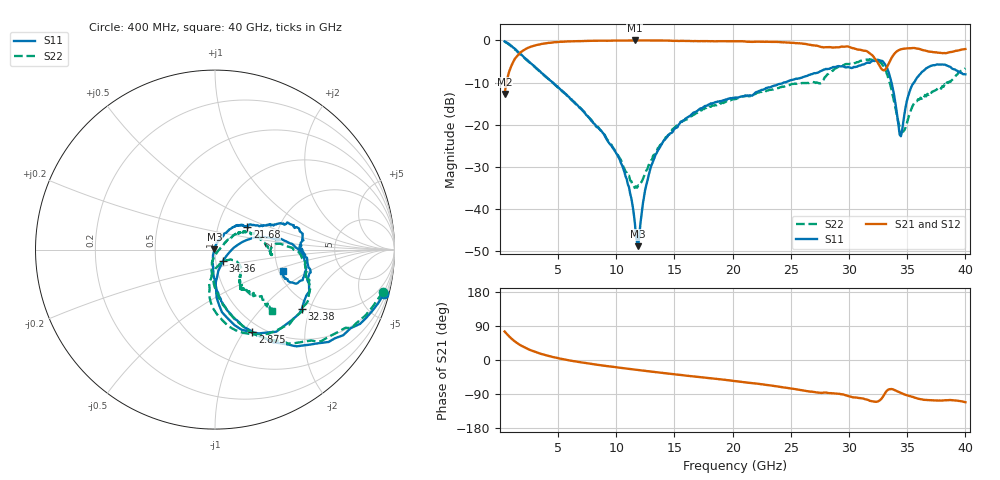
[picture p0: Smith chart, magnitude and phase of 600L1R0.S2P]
!  American Technical Ceramics  Date:  6/18/2004
!  One Norden Lane
!  Huntington Station,  NY.  11746-2102
!  Tel:  (631) 622-4700  Fax:  (631) 622-4748
!  Part Number  600L1R0  Mounting Orientation: Vertical
!  Description: Ultra Low ESR Microwave capacitors
!  Application: Coupling, Bypass, Tuning, DC Block
!  Filters, Matching
# GHZ S DB R 50
! Freq  |S11|  S11 Ph  |S21|  S21 Ph  |S12|  S12 Ph  |S22|  S22 Ph
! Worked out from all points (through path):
!   401 points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, 400 MHz to 40 GHz, reference 50 ohm
!   highest |S21| = 0.00 dB at 11.59 GHz (marker M1); lowest = -12.7 dB at 400 MHz (marker M2)
!   group delay of S21, straight-line fit = 10.3 ps
!   lowest |S11| = -48.9 dB at 11.88 GHz (marker M3), VSWR 1.01, Z = 49.7 + j0.152 ohm
!   |S11| at or under -10 dB: 4.537 GHz to 24.39 GHz (19.85 GHz wide, 137 % of centre); 33.65 GHz to 35.58 GHz (1.931 GHz wide, 5.58 % of centre)
!   |S22| runs from -35.0 to -0.3 dB; largest |S21 - S12| = 0.023
!   S11 on the Smith chart (normalised r, x): 400 MHz: 0.81, -7.73; 2.875 GHz: 0.89, -1.10; 21.68 GHz: 1.38, +0.37; 32.38 GHz: 1.76, -1.76; 34.36 GHz: 1.09, -0.13; 40 GHz: 2.10, -0.59
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0.4  -0.23 -14.6  -12.70 75.1  -12.78 75.2  -0.31 -14.2
1.291  -1.98 -40.6  -4.32 48.8  -4.40 48.3  -2.15 -40.8
2.875  -5.94 -65.7  -1.30 23.2  -1.30 23.4  -6.01 -66.6
7.033  -16.44 -92.2  -0.15 -6.5  -0.09 -6.4  -16.33 -96.0
10.3  -28.32 -107.1  -0.01 -20.4  0.00 -20.6  -27.96 -97.2
11.092  -34.86 -113.2  -0.02 -23.4  0.00 -23.6  -32.15 -75.5
11.587  -43.18 -136.3  0.00 -25.3  0.00 -25.4  -35.04 -47.1
11.884  -48.87 154.8  0.00 -26.4  0.00 -26.6  -34.44 -24.9
12.676  -33.31 82.1  -0.01 -29.4  -0.01 -29.6  -30.52 13.6
13.666  -25.76 68.0  -0.02 -33.0  0.00 -33.4  -25.34 30.3
16.636  -17.14 54.4  -0.16 -43.3  -0.19 -44.1  -17.67 37.3
20.2  -13.58 39.2  -0.18 -55.5  -0.30 -55.3  -13.92 28.5
21.685  -13.11 35.3  -0.34 -60.8  -0.43 -60.6  -12.90 23.4
26.833  -7.98 21.3  -1.14 -83.6  -1.15 -84.0  -9.79 -5.9
30.694  -6.23 -1.0  -2.13 -99.3  -2.14 -98.5  -5.15 -17.9
32.377  -4.65 -34.2  -4.89 -110.2  -4.86 -109.1  -4.75 -47.2
33.466  -8.13 -79.3  -5.15 -77.0  -5.15 -76.9  -9.78 -92.3
34.357  -22.39 -53.3  -2.20 -85.7  -2.20 -85.3  -20.63 -79.3
35.347  -11.06 14.6  -1.84 -96.4  -1.82 -95.9  -16.39 -30.2
36.436  -7.11 2.9  -2.35 -105.1  -2.34 -104.0  -13.59 -50.4
38.416  -5.99 -20.7  -2.96 -106.2  -2.92 -105.5  -9.97 -51.6
40  -8.05 -17.5  -2.03 -111.5  -1.94 -110.1  -6.62 -47.0
